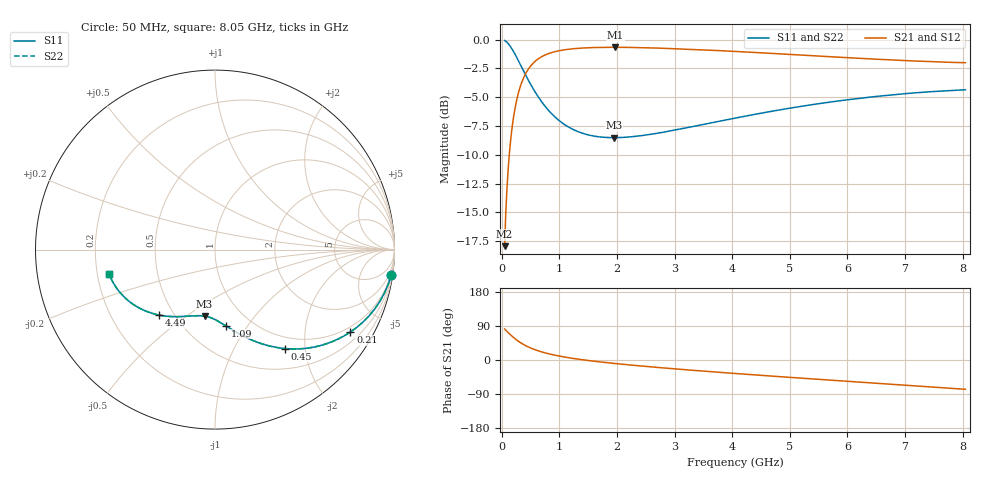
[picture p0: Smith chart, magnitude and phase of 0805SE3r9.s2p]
! AVX Thin Film Operation		Date: August 2001
! Description: Accu-P® Series, Thin Film, SMD, RF Capacitor
! Part Number: 08051J3R9ABT
! 50 MHz  -  8.05 GHz
! Serial Measurements
# mhz S db R 50
!	S11		S21		S12		S22
!	dB	Phase	dB	Phase	dB	Phase	dB	Phase
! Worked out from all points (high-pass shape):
!   401 points, 50 MHz to 8.05 GHz, reference 50 ohm
!   highest |S21| = -0.66 dB at 1.97 GHz (marker M1); lowest = -17.9 dB at 50 MHz (marker M2)
!   |S21| within 3 dB of the highest: 351.4 MHz to end of sweep
!   lowest |S11| = -8.5 dB at 1.95 GHz (marker M3), VSWR 2.20, Z = 34.2 - j29.5 ohm
!   |S11| at or under -10 dB: nowhere
!   |S22| runs from -8.5 to -0.1 dB; largest |S21 - S12| = 0
!   S11 on the Smith chart (normalised r, x): 50 MHz: 1, -14; 210 MHz: 0.81, -3.39; 450 MHz: 0.80, -1.63; 1.09 GHz: 0.77, -0.80; 4.49 GHz: 0.42, -0.40; 8.05 GHz: 0.25, -0.11
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50  -0.07 -8.1  -17.94 81.9  -17.94 81.9  -0.07 -8.1
90  -0.22 -14.4  -13.01 75.6  -13.01 75.6  -0.22 -14.4
110  -0.33 -17.4  -11.38 72.6  -11.38 72.6  -0.33 -17.4
130  -0.45 -20.4  -10.06 69.6  -10.06 69.6  -0.45 -20.4
170  -0.74 -26.1  -8.05 63.9  -8.05 63.9  -0.74 -26.1
210  -1.08 -31.3  -6.58 58.7  -6.58 58.7  -1.08 -31.3
310  -2.03 -42.7  -4.28 47.3  -4.28 47.3  -2.03 -42.7
450  -3.41 -54.7  -2.65 35.3  -2.65 35.3  -3.41 -54.7
570  -4.47 -62.4  -1.92 27.6  -1.92 27.6  -4.47 -62.4
710  -5.51 -69.3  -1.44 20.6  -1.44 20.6  -5.51 -69.3
890  -6.55 -76.2  -1.09 13.8  -1.09 13.8  -6.55 -76.2
1090  -7.38 -82.1  -0.88 7.9  -0.88 7.9  -7.38 -82.1
1390  -8.11 -89.0  -0.73 0.9  -0.73 0.9  -8.11 -89.0
1950  -8.52 -98.9  -0.66 -9.0  -0.66 -9.0  -8.52 -98.9
1970  -8.52 -99.2  -0.66 -9.3  -0.66 -9.3  -8.52 -99.2
2730  -8.11 -109.8  -0.73 -19.9  -0.73 -19.9  -8.11 -109.9
3370  -7.50 -117.7  -0.86 -27.8  -0.86 -27.8  -7.50 -117.7
4050  -6.82 -125.4  -1.02 -35.5  -1.02 -35.5  -6.82 -125.4
4490  -6.40 -130.3  -1.14 -40.4  -1.14 -40.4  -6.40 -130.3
5390  -5.65 -139.8  -1.39 -49.9  -1.39 -49.9  -5.65 -139.8
6730  -4.82 -153.5  -1.75 -63.7  -1.75 -63.7  -4.82 -153.5
8050  -4.36 -167.1  -2.01 -77.3  -2.01 -77.3  -4.36 -167.1
